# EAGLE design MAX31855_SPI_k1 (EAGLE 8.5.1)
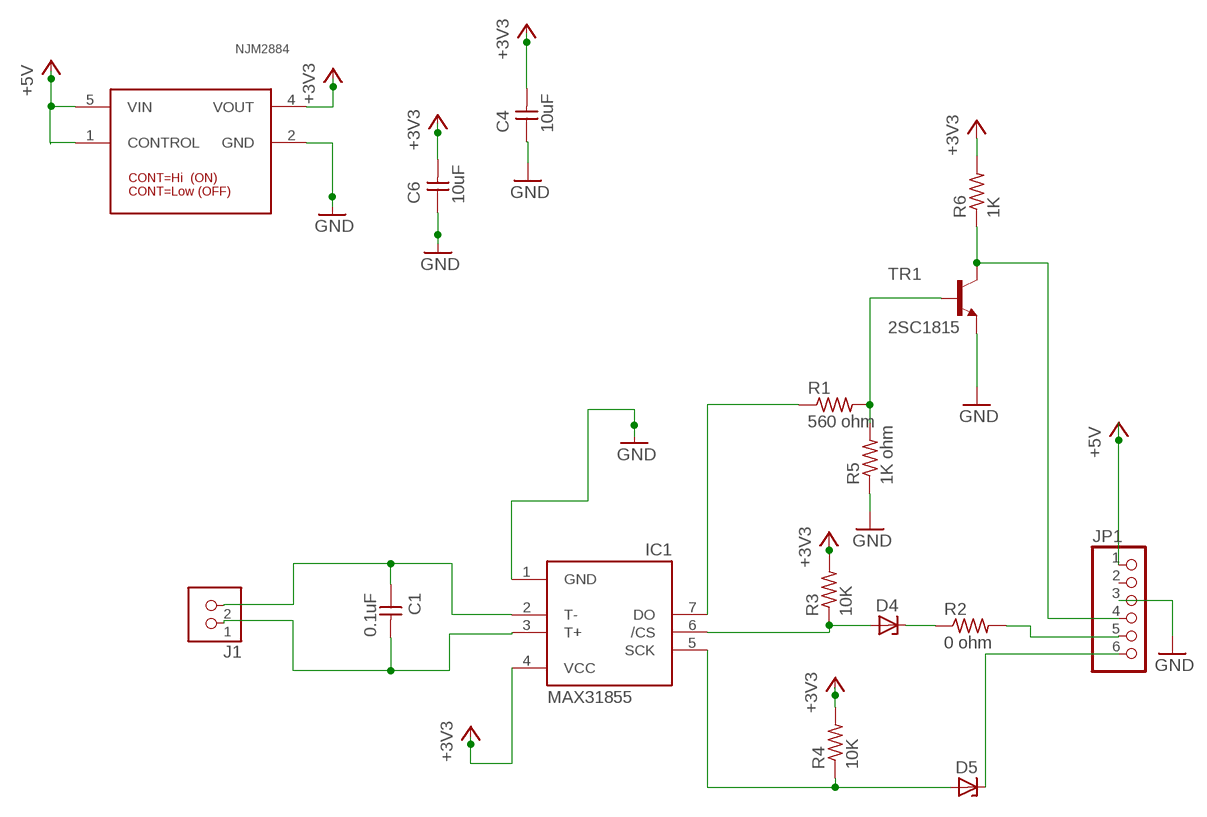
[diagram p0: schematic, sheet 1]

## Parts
C1  0.1uF  CAP-UNPOLARIZEDFAB  [C1206FAB]
C4  10uF  CAP-UNPOLARIZEDFAB  [C1206FAB]
C6  10uF  CAP-UNPOLARIZEDFAB  [C1206FAB]
D4  ZENER_DIODESOD123  [SOD123]
D5  ZENER_DIODESOD123  [SOD123]
IC1  MAX31855  MAX6675  [SO08]
J1  TERM-1X02-FABLAB  [ED555DS-2DS]
JP1  HEADER-1X676MIL  [1X06_ROUND_76]
NJM2884  I-10673_NJM2884U1-33  [NJM2884U1-33]
R1  560 ohm  RES-US1206FAB  [R1206FAB]
R2  0 ohm  RES-US1206FAB  [R1206FAB]
R3  10K  RES-US1206FAB  [R1206FAB]
R4  10K  RES-US1206FAB  [R1206FAB]
R5  1K ohm  RES-US1206FAB  [R1206FAB]
R6  1K  RES-US1206FAB  [R1206FAB]
TR1  2SC1815  I-06477_2SC1815  [TO92-BCE]

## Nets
+3V3: C4.2 C6.2 IC1.4(VCC) NJM2884.4(VOUT) R3.2 R4.2 R6.2
+5V: JP1.1 NJM2884.1(CONTROL) NJM2884.5(VIN)
CS: D4.ANODE IC1.6(/CS) R3.1
GND: C4.1 C6.1 IC1.1(GND) JP1.3 NJM2884.2(GND) R5.1 TR1.E
MISO: IC1.7(DO) R1.1
N$1: C1.1 IC1.2(T-) J1.2
N$2: D5.CATHODE JP1.6
N$3: JP1.5 R2.2
N$4: C1.2 IC1.3(T+) J1.1
N$5: R1.2 R5.2 TR1.B
N$6: JP1.4 R6.1 TR1.C
N$7: D4.CATHODE R2.1
SCK: D5.ANODE IC1.5(SCK) R4.1
Unconnected: JP1.2

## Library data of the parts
C1 C4 C6 = fab:CAP-UNPOLARIZED
D4 D5 = fab:ZENER_DIODE: zener diode
IC1 = adafruit:MAX6675
J1 = fab:TERM-1X02: 3.5mm terminal block, 2 positions ED555-2DS as found in the fablab inventory.
JP1 = microbuilder:HEADER-1X6: PIN HEADER
NJM2884 = Akizuki:I-10673_NJM2884U1-33
R1-R6 = fab:RES-US: Resistor (US Symbol)
TR1 = Akizuki:I-06477_2SC1815: NPN EPITAXIAL TRANSISTOR Source: TOSHIBA .. 2SC1815 1.pdf

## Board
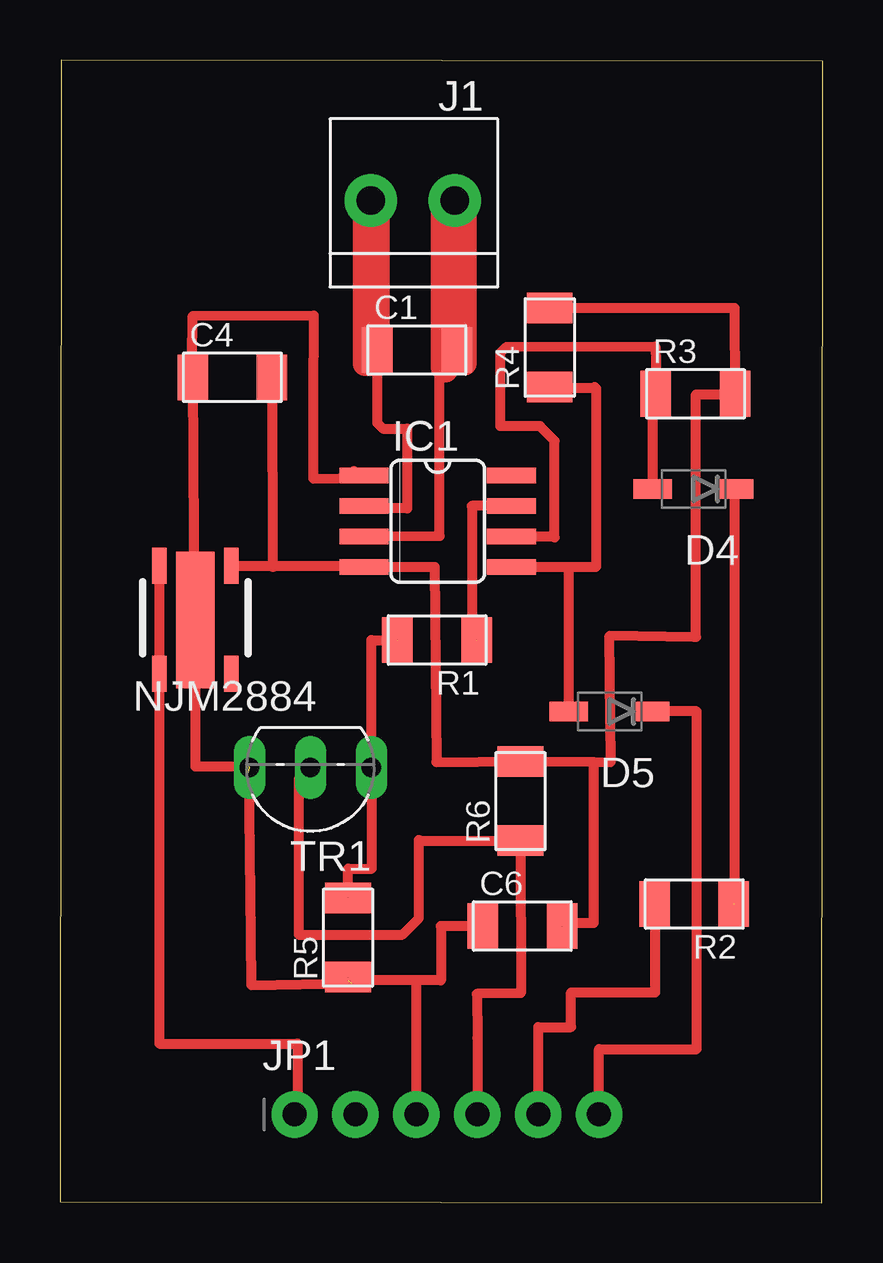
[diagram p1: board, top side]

Size 31.8 x 47.62 mm. Coordinates in mm from the lower left corner, seen from the top.
Outline: 0,0.05 31.75,0 31.8,47.56 0.05,47.61 0,0.05
Copper layers (1*16): Top 0.035mm / dielectric 1.5mm / Bottom 0.035mm
Design rules "default *": minimum track width 6mil, minimum drill 0.35mm, track to track 0.4mm, track to pad 0.4mm, pad to pad 0.4mm, via to via 0.4mm, smd to smd 0.4mm, copper to edge 40mil, drill to drill 6mil, minimum pad ring 10mil, minimum via ring 8mil, stop-mask expansion 4mil, vias tented up to drill 0mil, thermal gap 10mil

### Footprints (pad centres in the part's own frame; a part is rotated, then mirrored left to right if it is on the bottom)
C1206FAB = smd 1.27 x 1.905: 1 -1.651,0; 2 1.651,0
SOD123 = smd 1.6 x 0.8: ANODE 1.7,0; CATHODE -1.7,0
SO08 = smd 0.66 x 2.032: 1 -1.905,-3.073; 2 -0.635,-3.073; 3 0.635,-3.073; 4 1.905,-3.073; 5 1.905,3.073; 6 0.635,3.073; 7 -0.635,3.073; 8 -1.905,3.073
ED555DS-2DS = drill 1.2 pad 2.184: 1 1.8,0; 2 -1.7,0
1X06_ROUND_76 = drill 1 pad 1.93: 1 -6.35,0; 2 -3.81,0; 3 -1.27,0; 4 1.27,0; 5 3.81,0; 6 6.35,0
NJM2884U1-33 = smd 0.6 x 1.5: 1 -1.5,-2.25; 3 1.5,-2.25; 4 1.5,2.25; 5 -1.5,2.25 | smd 1.6 x 5.7: 2 0,0
R1206FAB = smd 1.27 x 1.905: 1 -1.651,0; 2 1.651,0
TO92-BCE = drill 0.813 long: B -2.54,0; C 0,0; E 2.54,0

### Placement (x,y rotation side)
C1  14.88,35.53 0 top
C4  7.19,34.39 0 top
C6  19.28,11.53 0 top
D4  26.42,29.74 180 top
D5  22.91,20.47 180 top
IC1  15.75,28.4 270 top
J1  14.66,41.76 0 top
JP1  16.13,3.68 0 top
NJM2884  5.64,24.28 0 top
R1  15.72,23.44 180 top
R2  26.44,12.45 180 top
R3  26.49,33.71 0 top
R4  20.42,35.64 90 top
R5  12.01,11.05 90 top
R6  19.2,16.74 90 top
TR1  10.44,18.14 180 top

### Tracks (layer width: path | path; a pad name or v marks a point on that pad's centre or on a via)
+3V3  (1 unrouted)
  Top 0.406: NJM2884.4 9.04,26.53 | 9.04,26.53 12.63,26.53 IC1.4 15.62,26.49 15.7,18.36 R6.2 22.25,18.37 | C4.2 8.87,26.49 9.04,26.53 | R4.2 28.12,37.29 R3.2 | R3.2 28.25,33.78 | 22.25,18.37 22.96,18.36 22.91,23.62 26.44,23.57 26.52,23.57 26.52,33.68 28.14,33.68 R3.2 | C6.2 20.93,11.66 22.25,11.66 22.25,18.37
+5V
  Top 0.406: NJM2884.5 NJM2884.1 4.14,6.63 9.91,6.63 9.91,3.68 JP1.1
CS
  Top 0.406: 24.93,33.62 24.72,33.4 24.72,33.71 R3.1 24.89,33.65 | IC1.6 20.57,27.76 20.62,27.71 20.62,31.75 20.02,32.36 18.36,32.36 18.36,35.41 18.62,35.66 24.82,35.69 24.89,33.65 | 24.89,33.65 24.93,33.62 | D4.ANODE 24.72,33.62 24.93,33.62
GND  (4 unrouted)
  Top 0.406: 12.24,30.48 12.06,30.3 | 12.01,30.25 12.06,30.3 | 12.06,30.3 IC1.1 12.68,30.2 10.56,30.17 10.56,33.44 10.58,36.98 5.54,36.96 5.51,35.1 C4.1 5.59,24.33 NJM2884.2 5.64,18.19 7.87,18.19 | 14.73,3.81 JP1.3 14.86,9.27 | 7.87,17.91 7.95,11.07 7.98,9.07 12.17,9.14 | C6.1 15.88,11.53 15.88,9.27 14.86,9.27 | 14.86,9.27 12.01,9.27 R5.1
MISO  (1 unrouted)
  Top 0.152: 18.16,29.03 IC1.7
  Top 0.406: 17.89,29.03 18.16,29.03 | IC1.7 17.17,29.03 17.17,23.44 R1.1
N$1
  Top 0.406: 13.44,35.74 C1.1 | IC1.2 12.78,28.93 14.48,28.93 14.48,32.26 13.46,32.26 13.23,32.49 13.23,39.06
  Top 1.016: 13.13,35 13.08,34.95 12.72,34.95 12.72,41.43 J1.2 13.23,41.58 13.23,39.06 C1.1
N$2
  Top 0.406: D5.CATHODE 26.54,20.47 26.54,10.52 26.54,10.16 26.54,6.4 22.48,6.4 JP1.6
N$3
  Top 0.406: JP1.5 19.94,7.31 21.31,7.31 21.31,8.76 24.82,8.76 24.82,12.45 R2.2
N$4
  Top 0.406: 12.7,27.74 IC1.3 15.82,27.79 15.82,34.62 16.08,34.7 16.08,35.08 C1.2 16.56,35.56 16.56,36.12
  Top 1.016: 16.56,36.12 J1.1 16.87,41.45 16.87,34.98 15.98,35.86 | 15.98,35.86 15.98,41.71 | 15.98,35.86 15.98,34.8 16.08,34.7
N$5  (3 unrouted)
  Top 0.406: R5.2 12.01,13.92 13.01,13.92 13.01,18.39 TR1.B 12.98,23.44 R1.2
N$6
  Top 0.406: JP1.4 17.4,6.86 17.38,8.7 19.21,8.73 R6.1 15.01,15.09 14.96,15.11 14.96,11.86 14.28,11.18 9.96,11.18 9.96,17.65 TR1.C
N$7  (1 unrouted)
  Top 0.406: D4.CATHODE 28.12,12.45 R2.1
SCK
  Top 0.406: 22.3,33.98 22.35,33.93 | 22.35,33.93 22.35,26.52 22.33,26.49 21.21,26.49 | 22.35,33.93 20.47,33.93 R4.1 | IC1.5 21.21,26.49 | D5.ANODE 21.21,26.49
